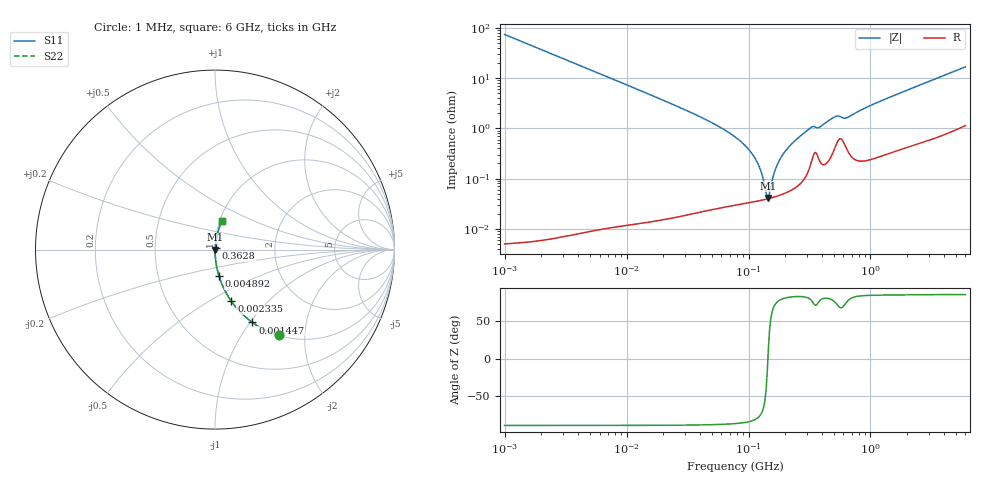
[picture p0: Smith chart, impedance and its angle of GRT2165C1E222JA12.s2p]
!Murata Part Number: GRT2165C1E222JA12
!These Parameters are Measured in Series Mode Connection
!Data Generated on Jun 19, 2026
!  o--ll--o
!Port1  Port2
!  o------o
!Operation Temp=25[degC], DC Bias Voltage=0[V]
!Freq. Start=1000[kHz] Stop=6[GHz] 401[Steps]
# Hz S RI R 50
!Freq.(Hz) S11(Real) S11(Imag) S21(Real) S21(Imag) S12(Real) S12(Imag) S22(Real) S22(Imag)
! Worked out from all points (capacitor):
!   401 points, 1 MHz to 6 GHz, reference 50 ohm
!   read as one part in series: C = 2.15 nF near 1.044 MHz
!   lowest |Z| = 41.1 mohm at 145.5 MHz (marker M1)
!   series resonance near 144.2 MHz, so ESL is about 570 pH
!   S11 on the Smith chart (normalised r, x): 1 MHz: 1.00, -1.48; 1.447 MHz: 1.00, -1.02; 2.335 MHz: 1.00, -0.63; 4.892 MHz: 1.00, -0.30; 362.8 MHz: 1.01, +0.02; 6 GHz: 1.02, +0.33
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1000000  0.3549 -0.4785  0.6451 0.4785  0.6451 0.4785  0.3549 -0.4785
1447343  0.208 -0.4058  0.792 0.4058  0.792 0.4058  0.208 -0.4058
2335446  0.0916 -0.2884  0.9084 0.2884  0.9084 0.2884  0.0916 -0.2884
4293785  0.029 -0.1675  0.971 0.1675  0.971 0.1675  0.029 -0.1675
4892295  0.0225 -0.148  0.9775 0.148  0.9775 0.148  0.0225 -0.148
1.843659e7  0.0017 -0.0394  0.9983 0.0394  0.9983 0.0394  0.0017 -0.0394
4.596069e7  0.000438 -0.0144  0.9996 0.0144  0.9996 0.0144  0.000438 -0.0144
7.745967e7  0.00034 -0.00677  0.9997 0.00677  0.9997 0.00677  0.00034 -0.00677
9.627852e7  0.000341 -0.00424  0.9997 0.00424  0.9997 0.00424  0.000341 -0.00424
1.121107e8  0.000353 -0.0026  0.9996 0.0026  0.9996 0.0026  0.000353 -0.0026
1.249896e8  0.000368 -0.00147  0.9996 0.00147  0.9996 0.00147  0.000368 -0.00147
1.39348e8  0.000388 -0.000349  0.9996 0.000349  0.9996 0.000349  0.000388 -0.000349
1.455431e8  0.000398 9.84e-05  0.9996 -9.84e-05  0.9996 -9.84e-05  0.000398 9.84e-05
1.658303e8  0.000437 0.00145  0.9996 -0.00145  0.9996 -0.00145  0.000437 0.00145
1.889453e8  0.000493 0.00284  0.9995 -0.00284  0.9995 -0.00284  0.000493 0.00284
2.348496e8  0.000654 0.00535  0.9993 -0.00535  0.9993 -0.00535  0.000654 0.00535
3.325952e8  0.00253 0.0104  0.9975 -0.0104  0.9975 -0.0104  0.00253 0.0104
3.628252e8  0.00316 0.00979  0.9968 -0.00979  0.9968 -0.00979  0.00316 0.00979
5.138348e8  0.0045 0.0165  0.9955 -0.0165  0.9955 -0.0165  0.0045 0.0165
6.386712e8  0.00411 0.0157  0.9959 -0.0157  0.9959 -0.0157  0.00411 0.0157
1.428092e9  0.00485 0.041  0.9951 -0.041  0.9951 -0.041  0.00485 0.041
6e9  0.0376 0.1593  0.9624 -0.1593  0.9624 -0.1593  0.0376 0.1593
